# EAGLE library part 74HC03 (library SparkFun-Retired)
Quad 2-input open-drain NAND 2-5V operating voltage Some part numbers may include a clamping diode from OD output to VCC; check datasheet for specific part. We use an NXP part which does NOT have a clamping diode. Doesn't seem to be in inventory anywhere. We have nands but not open-drain
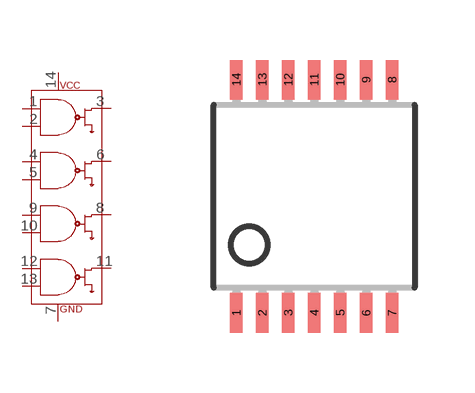
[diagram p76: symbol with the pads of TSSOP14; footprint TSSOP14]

Designator prefix -

## 74HC03  [TSSOP14]
1  A1
2  B1
3  Y1
4  A2
5  B2
6  Y2
7  VSS
8  Y3
9  A3
10  B3
11  Y4
12  A4
13  B4
14  VCC

## Footprint TSSOP14 (pad centres in mm)
Thin Shrink Small Outline Plastic 14
smd 0.305 x 0.991: 1 -1.95,-2.918; 2 -1.3,-2.918; 3 -0.65,-2.918; 4 0,-2.918; 5 0.65,-2.918; 6 1.3,-2.918; 7 1.95,-2.918; 8 1.95,2.918; 9 1.3,2.918; 10 0.65,2.918; 11 0,2.918; 12 -0.65,2.918; 13 -1.3,2.918; 14 -1.95,2.918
